| IBIS file stm32u375_385_ufbga100_smps.ibs
[IBIS ver] 4.2
[File name] stm32u375_385_ufbga100_smps.ibs
[File Rev] 1.2
[Date] 23-06-2025
[Source] Data Created at STMicroelectronics
[Notes]  File originated from ELDO simulations.
[Disclaimer]  This information is for modeling purpose only and is
   not guaranted. The information is subject to change without
   notice.
[Copyright] Copyright 2025 STMicroelectronics Inc.
|   Component stm32u375_385_ufbga100_smps
[Component] stm32u375_385_ufbga100_smps
[Manufacturer] STMicroelectronics
[Package]
| variable   typ   min   max
R_pkg  0  NA  NA
L_pkg  0  NA  NA
C_pkg  0  NA  NA
[Pin]   signal_name   model_name
A1  PB9  io8_ft_100m_hslv
A2  PE0  io8_ft_100m
A3  PH3-BOOT0  io8_ft_100m_hslv
A4  PB7  io8_ft_100m_hslv
A5  PB6  io8_ft_100m_hslv
A6  PB4  io8_ft_100m_hslv
A7  PD7  io8_ft_100m_hslv
A8  PD5  io8_ft_100m_hslv
A9  PD4  io8_ft_100m_hslv
A10  PD2  io8_ft_100m_hslv
A11  PD0  io8_ft_100m
A12  PC10  io8_ft_100m_hslv
B1  PE2  io8_ft_100m
B2  PE3  io8_ft_100m_hslv
B3  PE4  io8_ft_100m
B4  PB8  io8_ft_100m_hslv
B5  PB5  io8_ft_100m_hslv
B6  PB3  io8_ft_100m_hslv
B7  VDD  power
B8  PD6  io8_ft_100m_hslv
B9  PD3  io8_ft_100m_hslv
B10  PD1  io8_ft_100m
B11  PC11  io8_ft_100m_hslv
B12  PA15  io8_ft_100m
C1  VBAT  power
C2  PE6  io8_ft_100m
C3  VDD  power
C4  VSS  gnd
C5  VDD11  nc
C8  VSS  gnd
C9  PC12  io8_ft_100m_hslv
C10  VDD  power
C11  PA14  io8_ft_100m
C12  PA13  io8_ft_100m
D1  PC14-OSC32_IN  io_ft_tamp
D2  PC15-OSC32_OUT  io_ft_tamp
D3  PE5  io8_ft_100m
D10  VSS  gnd
D11  PA12  io8usb_ft_phy
D12  PA11  io8usb_ft_phy
E1  PH0-OSC_IN  io8_ft_100m
E2  PH1-OSC_OUT  io8_ft_100m
E3  PC13  io8_ft_100m_v33
E10  VDDUSB  power
E11  PA9  io8_ft_100m
E12  PA10  io8_ft_100m
F1  NRST  ioreset_v33
F2  PC0  io8_ft_100m_hslv
F11  PC9  io8_ft_100m_hslv
F12  PA8  io8_ft_100m_hslv
G1  PC1  io8_ft_100m_hslv
G2  PC2  io8_ft_100m_hslv
G11  PC7  io8_ft_100m_hslv
G12  PC8  io8_ft_100m_hslv
H1  VREFP  nc
H2  VSSA  nc
H3  PC3  io8_ft_100m_hslv
H10  PD12  io8_ft_100m_hslv
H11  PD15  io8_ft_100m
H12  PC6  io8_ft_100m_hslv
J1  VDDA  nc
J2  PA1  io8_ft_100m_hslv
J3  PA0  io8_ft_100m
J10  PD8  io8_ft_100m
J11  PD13  io8_ft_100m_hslv
J12  PD14  io8_ft_100m
K1  PA2  io8_ft_100m_hslv
K2  PA3  io8_ft_100m_hslv
K3  VSS  gnd
K4  VDD  power
K5  PE7  io8_ft_100m
K8  PB11  io8_ft_100m_hslv
K9  VDD11  nc
K10  VDD  power
K11  PD9  io8_ft_100m
K12  PD11  io8_ft_100m
L1  PA4  io8_ft_100m_hslv
L2  PA5  io8_ft_100m
L3  PB0  io8_ft_100m_hslv
L4  PB2  io8_ft_100m_hslv
L5  PE9  io8_ft_100m_hslv
L6  PE11  io8_ft_100m_hslv
L7  PE13  io8_ft_100m_hslv
L8  PE15  io8_ft_100m_hslv
L9  VSSSMPS  nc
L10  VSS  gnd
L11  PB13  io8_ft_100m_hslv
L12  PD10  io8_ft_100m
M1  PA6  io8_ft_100m_hslv
M2  PA7  io8_ft_100m_hslv
M3  PB1  io8_ft_100m_hslv
M4  PE8  io8_ft_100m
M5  PE10  io8_ft_100m_hslv
M6  PE12  io8_ft_100m_hslv
M7  PE14  io8_ft_100m_hslv
M8  PB10  io8_ft_100m_hslv
M9  VLXSMPS  nc
M10  VDDSMPS  nc
M11  PB14  io8_ft_100m_hslv
M12  PB15  io8_ft_100m
[Package Model]   454-ufbga-7x7-100-smps-250417
[Pin Mapping]   pulldown_ref   pullup_ref   | Comment
A1  gndio  vddio
A2  gndio  vddio
A3  gndio  vddio
A4  gndio  vddio
A5  gndio  vddio
A6  gndio  vddio
A7  gndio  vddio
A8  gndio  vddio
A9  gndio  vddio
A10  gndio  vddio
A11  gndio  vddio
A12  gndio  vddio
B1  gndio  vddio
B2  gndio  vddio
B3  gndio  vddio
B4  gndio  vddio
B5  gndio  vddio
B6  gndio  vddio
B7  nc  vddio
B8  gndio  vddio
B9  gndio  vddio
B10  gndio  vddio
B11  gndio  vddio
B12  gndio  vddio
C1  nc  vsw
C2  gndio  vddio
C3  nc  vddio
C4  gndio  nc
C5  nc  nc
C8  gndio  nc
C9  gndio  vddio
C10  nc  vddio
C11  gndio  vddio
C12  gndio  vddio
D1  gndio  vsw
D2  gndio  vsw
D3  gndio  vddio
D10  gndio  nc
D11  gndio  vddusb  | Depending on IO usage
| D11  gndio  vddio  | Depending on IO usage
D12  gndio  vddusb  | Depending on IO usage
| D12  gndio  vddio  | Depending on IO usage
E1  gndio  vddio
E2  gndio  vddio
E3  gndio  vsw
E10  nc  vddusb
E11  gndio  vddio
E12  gndio  vddio
F1  gndio  vddio
F2  gndio  vddio
F11  gndio  vddio
F12  gndio  vddio
G1  gndio  vddio
G2  gndio  vddio
G11  gndio  vddio
G12  gndio  vddio
H1  nc  nc
H2  nc  nc
H3  gndio  vddio
H10  gndio  vddio
H11  gndio  vddio
H12  gndio  vddio
J1  nc  nc
J2  gndio  vddio
J3  gndio  vddio
J10  gndio  vddio
J11  gndio  vddio
J12  gndio  vddio
K1  gndio  vddio
K2  gndio  vddio
K3  gndio  nc
K4  nc  vddio
K5  gndio  vddio
K8  gndio  vddio
K9  nc  nc
K10  nc  vddio
K11  gndio  vddio
K12  gndio  vddio
L1  gndio  vddio
L2  gndio  vddio
L3  gndio  vddio
L4  gndio  vddio
L5  gndio  vddio
L6  gndio  vddio
L7  gndio  vddio
L8  gndio  vddio
L9  nc  nc
L10  gndio  nc
L11  gndio  vddio
L12  gndio  vddio
M1  gndio  vddio
M2  gndio  vddio
M3  gndio  vddio
M4  gndio  vddio
M5  gndio  vddio
M6  gndio  vddio
M7  gndio  vddio
M8  gndio  vddio
M9  nc  nc
M10  nc  nc
M11  gndio  vddio
M12  gndio  vddio
|[Diff Pin]  inv_pin  vdiff  tdelay_typ  tdelay_min  tdelay_max
|D11  D12  NA  NA  NA  NA
[Model Selector] io8_ft_100m
io8_ft_100m_ls_1v2  "GPIO 100MHz - 5V tolerant - low speed - 1.2V range"
io8_ft_100m_ls_1v8  "GPIO 100MHz - 5V tolerant - low speed - 1.8V range"
io8_ft_100m_ls_3v3  "GPIO 100MHz - 5V tolerant - low speed - 3.3V range"
io8_ft_100m_ms_1v2  "GPIO 100MHz - 5V tolerant - med speed - 1.2V range"
io8_ft_100m_ms_1v8  "GPIO 100MHz - 5V tolerant - med speed - 1.8V range"
io8_ft_100m_ms_3v3  "GPIO 100MHz - 5V tolerant - med speed - 3.3V range"
io8_ft_100m_fs_1v2  "GPIO 100MHz - 5V tolerant - fast speed - 1.2V range"
io8_ft_100m_fs_1v8  "GPIO 100MHz - 5V tolerant - fast speed - 1.8V range"
io8_ft_100m_fs_3v3  "GPIO 100MHz - 5V tolerant - fast speed - 3.3V range"
io8_ft_100m_hs_1v2  "GPIO 100MHz - 5V tolerant - high speed - 1.2V range"
io8_ft_100m_hs_1v8  "GPIO 100MHz - 5V tolerant - high speed - 1.8V range"
io8_ft_100m_hs_3v3  "GPIO 100MHz - 5V tolerant - high speed - 3.3V range"
[Model Selector] io8_ft_100m_hslv
io8_ft_100m_ls_1v2  "GPIO 100MHz - 5V tolerant - low speed - 1.2V range"
io8_ft_100m_ls_1v8  "GPIO 100MHz - 5V tolerant - low speed - 1.8V range"
io8_ft_100m_ls_3v3  "GPIO 100MHz - 5V tolerant - low speed - 3.3V range"
io8_ft_100m_ms_1v2  "GPIO 100MHz - 5V tolerant - med speed - 1.2V range"
io8_ft_100m_ms_1v8  "GPIO 100MHz - 5V tolerant - med speed - 1.8V range"
io8_ft_100m_ms_3v3  "GPIO 100MHz - 5V tolerant - med speed - 3.3V range"
io8_ft_100m_fs_1v2  "GPIO 100MHz - 5V tolerant - fast speed - 1.2V range"
io8_ft_100m_fs_1v8  "GPIO 100MHz - 5V tolerant - fast speed - 1.8V range"
io8_ft_100m_fs_3v3  "GPIO 100MHz - 5V tolerant - fast speed - 3.3V range"
io8_ft_100m_hs_1v2  "GPIO 100MHz - 5V tolerant - high speed - 1.2V range"
io8_ft_100m_hs_1v8  "GPIO 100MHz - 5V tolerant - high speed - 1.8V range"
io8_ft_100m_hs_3v3  "GPIO 100MHz - 5V tolerant - high speed - 3.3V range"
io8_ft_100m_hslv_ls_1v2  "GPIO 100MHz low voltage optimization - 5V tolerant - low speed - 1.2V range"
io8_ft_100m_hslv_ls_1v8  "GPIO 100MHz low voltage optimization - 5V tolerant - low speed - 1.8V range"
io8_ft_100m_hslv_ls_2v5  "GPIO 100MHz low voltage optimization - 5V tolerant - low speed - 3.3V range"
io8_ft_100m_hslv_ms_1v2  "GPIO 100MHz low voltage optimization - 5V tolerant - med speed - 1.2V range"
io8_ft_100m_hslv_ms_1v8  "GPIO 100MHz low voltage optimization - 5V tolerant - med speed - 1.8V range"
io8_ft_100m_hslv_ms_2v5  "GPIO 100MHz low voltage optimization - 5V tolerant - med speed - 3.3V range"
io8_ft_100m_hslv_fs_1v2  "GPIO 100MHz low voltage optimization - 5V tolerant - fast speed - 1.2V range"
io8_ft_100m_hslv_fs_1v8  "GPIO 100MHz low voltage optimization - 5V tolerant - fast speed - 1.8V range"
io8_ft_100m_hslv_fs_2v5  "GPIO 100MHz low voltage optimization - 5V tolerant - fast speed - 3.3V range"
io8_ft_100m_hslv_hs_1v2  "GPIO 100MHz low voltage optimization - 5V tolerant - high speed - 1.2V range"
io8_ft_100m_hslv_hs_1v8  "GPIO 100MHz low voltage optimization - 5V tolerant - high speed - 1.8V range"
io8_ft_100m_hslv_hs_2v5  "GPIO 100MHz low voltage optimization - 5V tolerant - high speed - 3.3V range"
[Model Selector] io8_ft_100m_v33
io8_ft_100m_v33_ls_1v2  "GPIO_V33 100MHz - 5V tolerant - low speed - 1.2V range"
io8_ft_100m_v33_ls_1v8  "GPIO_V33 100MHz - 5V tolerant - low speed - 1.8V range"
io8_ft_100m_v33_ls_3v3  "GPIO_V33 100MHz - 5V tolerant - low speed - 3.3V range"
io8_ft_100m_v33_ms_1v2  "GPIO_V33 100MHz - 5V tolerant - med speed - 1.2V range"
io8_ft_100m_v33_ms_1v8  "GPIO_V33 100MHz - 5V tolerant - med speed - 1.8V range"
io8_ft_100m_v33_ms_3v3  "GPIO_V33 100MHz - 5V tolerant - med speed - 3.3V range"
io8_ft_100m_v33_fs_1v2  "GPIO_V33 100MHz - 5V tolerant - fast speed - 1.2V range"
io8_ft_100m_v33_fs_1v8  "GPIO_V33 100MHz - 5V tolerant - fast speed - 1.8V range"
io8_ft_100m_v33_fs_3v3  "GPIO_V33 100MHz - 5V tolerant - fast speed - 3.3V range"
io8_ft_100m_v33_hs_1v2  "GPIO_V33 100MHz - 5V tolerant - high speed - 1.2V range"
io8_ft_100m_v33_hs_1v8  "GPIO_V33 100MHz - 5V tolerant - high speed - 1.8V range"
io8_ft_100m_v33_hs_3v3  "GPIO_V33 100MHz - 5V tolerant - high speed - 3.3V range"
[Model Selector] io8usb_ft_phy
io8_ft_100m_ls_1v2  "GPIO 100MHz - 5V tolerant - low speed - 1.2V range"
io8_ft_100m_ls_1v8  "GPIO 100MHz - 5V tolerant - low speed - 1.8V range"
io8_ft_100m_ls_3v3  "GPIO 100MHz - 5V tolerant - low speed - 3.3V range"
io8_ft_100m_ms_1v2  "GPIO 100MHz - 5V tolerant - med speed - 1.2V range"
io8_ft_100m_ms_1v8  "GPIO 100MHz - 5V tolerant - med speed - 1.8V range"
io8_ft_100m_ms_3v3  "GPIO 100MHz - 5V tolerant - med speed - 3.3V range"
io8_ft_100m_fs_1v2  "GPIO 100MHz - 5V tolerant - fast speed - 1.2V range"
io8_ft_100m_fs_1v8  "GPIO 100MHz - 5V tolerant - fast speed - 1.8V range"
io8_ft_100m_fs_3v3  "GPIO 100MHz - 5V tolerant - fast speed - 3.3V range"
io8_ft_100m_hs_1v2  "GPIO 100MHz - 5V tolerant - high speed - 1.2V range"
io8_ft_100m_hs_1v8  "GPIO 100MHz - 5V tolerant - high speed - 1.8V range"
io8_ft_100m_hs_3v3  "GPIO 100MHz - 5V tolerant - high speed - 3.3V range"
io8usb_ft_phy_hs_3v3   "USB full speed"
io8usb_ft_phy_ls_3v3   "USB low speed"
[Model Selector] io_ft_tamp
io_ft_tamp_ls_1v2 "io8_ft tamp low speed @ 1.2V"
io_ft_tamp_ls_1v8 "io8_ft tamp low speed @ 1.8V"
io_ft_tamp_ls_3v3 "io8_ft tamp low speed @ 3.3V"
io_ft_tamp_ms_1v2 "io8_ft tamp med speed @ 1.2V"
io_ft_tamp_ms_1v8 "io8_ft tamp med speed @ 1.8V"
io_ft_tamp_ms_3v3 "io8_ft tamp med speed @ 3.3V"
io_ft_tamp_fs_1v2 "io8_ft tamp fast speed @ 1.2V"
io_ft_tamp_fs_1v8 "io8_ft tamp fast speed @ 1.8V"
io_ft_tamp_fs_3v3 "io8_ft tamp fast speed @ 3.3V"
io_ft_tamp_hs_1v2 "io8_ft tamp high speed @ 1.2V"
io_ft_tamp_hs_1v8 "io8_ft tamp high speed @ 1.8V"
io_ft_tamp_hs_3v3 "io8_ft tamp high speed @ 3.3V"
[Model Selector] ioreset_v33
ioreset_v33_1v2 "Reset PAD. 5V tolerant. 1.2V range"
ioreset_v33_1v8 "Reset PAD. 5V tolerant. 1.8V range"
ioreset_v33_3v3 "Reset PAD. 5V tolerant. 3.3V range"
[Define Package Model]  454-ufbga-7x7-100-smps-250417
[Manufacturer]  unknown
[OEM]  unknown
[Description]  unknown
[Number Of Pins]  92
[Pin Numbers]
| Pin Name Terminal   Net Name   Starting Node   Ending Node
F1 | NRST
J3 | PA0
J2 | PA1
K1 | PA2
K2 | PA3
L1 | PA4
L2 | PA5
M1 | PA6
M2 | PA7
F12 | PA8
E11 | PA9
E12 | PA10
D12 | PA11
D11 | PA12
C12 | PA13
C11 | PA14
B12 | PA15
L3 | PB0
M3 | PB1
L4 | PB2
B6 | PB3
A6 | PB4
B5 | PB5
A5 | PB6
A4 | PB7
B4 | PB8
A1 | PB9
M8 | PB10
K8 | PB11
L11 | PB13
M11 | PB14
M12 | PB15
F2 | PC0
G1 | PC1
G2 | PC2
H3 | PC3
H12 | PC6
G11 | PC7
G12 | PC8
F11 | PC9
A12 | PC10
B11 | PC11
C9 | PC12
E3 | PC13
D1 | PC14-OSC32_IN
D2 | PC15-OSC32_OUT
A11 | PD0
B10 | PD1
A10 | PD2
B9 | PD3
A9 | PD4
A8 | PD5
B8 | PD6
A7 | PD7
J10 | PD8
K11 | PD9
L12 | PD10
K12 | PD11
H10 | PD12
J11 | PD13
J12 | PD14
H11 | PD15
A2 | PE0
B1 | PE2
B2 | PE3
B3 | PE4
D3 | PE5
C2 | PE6
K5 | PE7
M4 | PE8
L5 | PE9
M5 | PE10
L6 | PE11
M6 | PE12
L7 | PE13
M7 | PE14
L8 | PE15
E1 | PH0-OSC_IN
E2 | PH1-OSC_OUT
A3 | PH3-BOOT0
K9 | VDD11
C5 | VDD11
C1 | VBAT
B7 | VDD
J1 | VDDA
M10 | VDDSMPS
E10 | VDDUSB
M9 | VLXSMPS
H1 | VREFP
C4 | VSS
H2 | VSSA
L9 | VSSSMPS
|[Merged Pins]  B7
|C3  |  VDD
|C10  |  VDD
|K4  |  VDD
|K10  |  VDD
|[Merged Pins]  C4
|C8  |  VSS
|D10  |  VSS
|K3  |  VSS
|L10  |  VSS
[Model Data]
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[End Model Data]
[End Package Model]
|End [Component]
| Models and submodels in the file (53): io8_ft_100m_fs_1v2 (I/O), io8_ft_100m_fs_1v8 (I/O), io8_ft_100m_fs_3v3 (I/O), io8_ft_100m_hs_1v2 (I/O), io8_ft_100m_hs_1v8 (I/O), io8_ft_100m_hs_3v3 (I/O), io8_ft_100m_hslv_fs_1v2 (I/O), io8_ft_100m_hslv_fs_1v8 (I/O), io8_ft_100m_hslv_fs_2v5 (I/O), io8_ft_100m_hslv_hs_1v2 (I/O), io8_ft_100m_hslv_hs_1v8 (I/O), io8_ft_100m_hslv_hs_2v5 (I/O), io8_ft_100m_hslv_ls_1v2 (I/O), io8_ft_100m_hslv_ls_1v8 (I/O), io8_ft_100m_hslv_ls_2v5 (I/O), io8_ft_100m_hslv_ms_1v2 (I/O), io8_ft_100m_hslv_ms_1v8 (I/O), io8_ft_100m_hslv_ms_2v5 (I/O), io8_ft_100m_ls_1v2 (I/O), io8_ft_100m_ls_1v8 (I/O), io8_ft_100m_ls_3v3 (I/O), io8_ft_100m_ms_1v2 (I/O), io8_ft_100m_ms_1v8 (I/O), io8_ft_100m_ms_3v3 (I/O), io8_ft_100m_v33_fs_1v2 (I/O), io8_ft_100m_v33_fs_1v8 (I/O), io8_ft_100m_v33_fs_3v3 (I/O), io8_ft_100m_v33_hs_1v2 (I/O), io8_ft_100m_v33_hs_1v8 (I/O), io8_ft_100m_v33_hs_3v3 (I/O), io8_ft_100m_v33_ls_1v2 (I/O), io8_ft_100m_v33_ls_1v8 (I/O), io8_ft_100m_v33_ls_3v3 (I/O), io8_ft_100m_v33_ms_1v2 (I/O), io8_ft_100m_v33_ms_1v8 (I/O), io8_ft_100m_v33_ms_3v3 (I/O), io8usb_ft_phy_hs_3v3 (I/O), io8usb_ft_phy_ls_3v3 (I/O), io_ft_tamp_fs_1v2 (I/O), io_ft_tamp_fs_1v8 (I/O), io_ft_tamp_fs_3v3 (I/O), io_ft_tamp_hs_1v2 (I/O), io_ft_tamp_hs_1v8 (I/O), io_ft_tamp_hs_3v3 (I/O), io_ft_tamp_ls_1v2 (I/O), io_ft_tamp_ls_1v8 (I/O), io_ft_tamp_ls_3v3 (I/O), io_ft_tamp_ms_1v2 (I/O), io_ft_tamp_ms_1v8 (I/O), io_ft_tamp_ms_3v3 (I/O), ioreset_v33_1v2 (I/O_open_drain), ioreset_v33_1v8 (I/O_open_drain), ioreset_v33_3v3 (I/O_open_drain)
